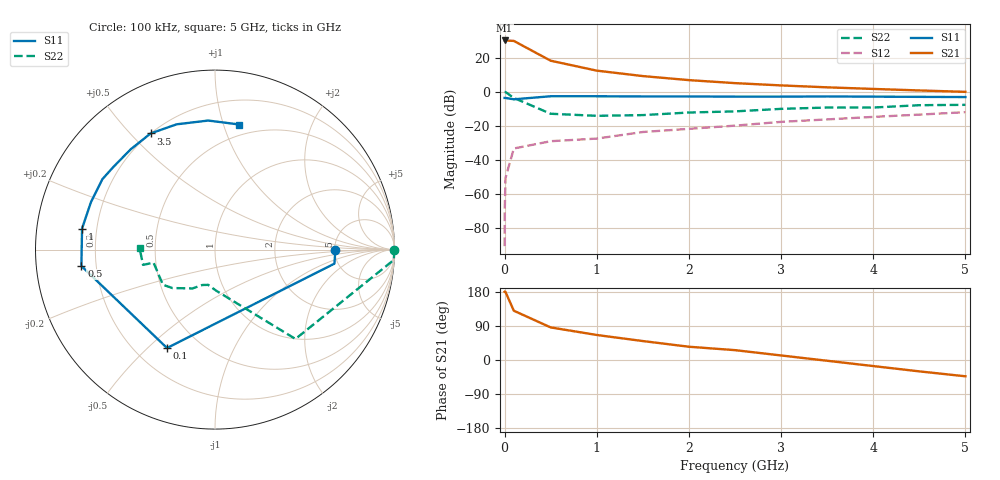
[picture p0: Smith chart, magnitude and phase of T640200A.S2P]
!AT-64020
!S-PARAMETERS at Vce=16V  Ic=110mA.  LAST UPDATED 07-21-92
# ghz s ma r 50
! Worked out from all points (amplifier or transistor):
!   14 points, 100 kHz to 5 GHz, reference 50 ohm
!   highest |S21| = 30.2 dB at 100 kHz (marker M1)
!   |S21| within 3 dB of that: start of sweep to 194 MHz
!   unconditionally stable (mu >= 1): 850 MHz to 3.005 GHz
!   at 10 MHz: K = -0.02, MSG = 40.3 dB, |S12| = -50.5 dB
!   at 2 GHz: K = 1.13, MAG = 12.1 dB, |S12| = -21.6 dB
!   at 5 GHz: K = 0.80, MSG = 6.0 dB, |S12| = -11.8 dB
!   S11 on the Smith chart (normalised r, x): 100 kHz: 5.06, -0.02; 100 MHz: 0.33, -0.58; 500 MHz: 0.14, -0.06; 1 GHz: 0.14, +0.08; 3.5 GHz: 0.20, +0.57; 5 GHz: 0.40, +1.13
0.0001  0.67 -0.1  32.5 179.9  3e-05 88.0  0.999 0.0
0.001  0.67 -0.7  32.5 179.6  0.0003 89.0  0.999 -0.3
0.01  0.67 -6.7  32.4 179.5  0.003 87.0  0.998 -3.3
0.1  0.61 -116.0  31.51 130.0  0.022 57.0  0.67 -48.0
0.5  0.75 -173.0  8.27 86.0  0.036 41.0  0.23 -88.0
1  0.75 171.0  4.23 66.0  0.043 49.0  0.2 -101.0
1.5  0.74 159.0  2.93 50.0  0.067 48.0  0.21 -110.0
2  0.74 148.0  2.23 35.0  0.083 46.0  0.25 -120.0
2.5  0.73 141.0  1.82 26.0  0.103 47.0  0.27 -127.0
3  0.73 130.0  1.56 12.0  0.133 41.0  0.32 -138.0
3.5  0.74 119.0  1.37 -2.0  0.157 35.0  0.35 -146.0
4  0.73 107.0  1.23 -16.0  0.186 26.0  0.35 -168.0
4.5  0.72 93.0  1.11 -30.0  0.217 18.0  0.41 -168.0
5  0.71 79.0  1.01 -43.0  0.256 8.0  0.42 179.0
